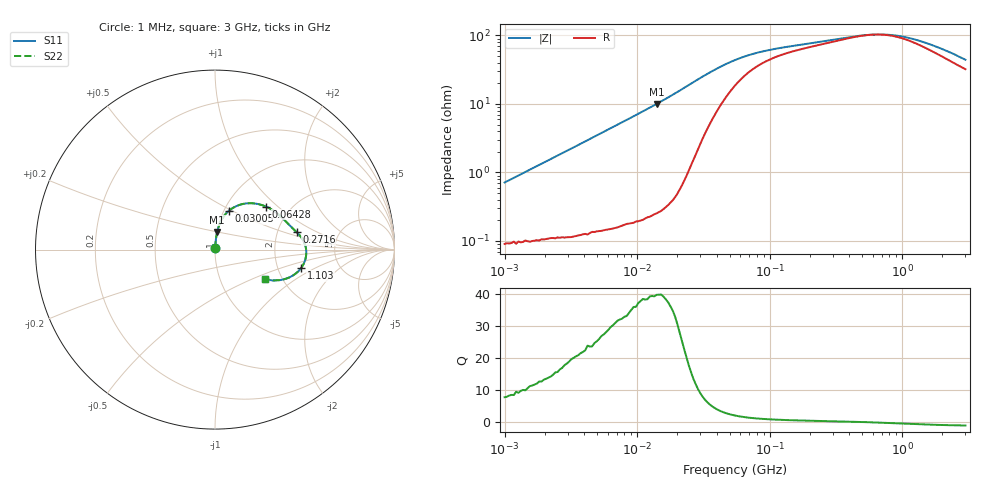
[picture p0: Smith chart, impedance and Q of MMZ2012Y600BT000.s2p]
! S-parameter Generated by TDK Corporation
! Copyright(C) 2016 TDK Corporation.
! All Rights Reserved.
! TDK P/N: MMZ2012Y600BT000 (Chip Beads)
! Property: |Z|=60¶ at 100MHz
! Size(LxWxT): 2x1.25x0.85mm, 0.079x0.049x0.033inches
! Model Type: s2p (Touchstone File Format Version 1.0)
! Frequency: DC=Yes Start=1MHz Stop=3000MHz 202points Log-sweep
! Note: This model was converted from impedance.
! Model Generated on May. 16, 2016
! Hash(MD5):
! Port Assignments:
!  1 ---@@@--- 2
! Applicable Conditions:
!  Temperature = 25 degC
!  DC Bias Current = 0 A
!  Small Signal Operation
! Terms and conditions regarding TDK Simulation Models
! (1)This simulation model is being provided solely for informational purposes. Please refer to the specifications of the products in terms of detailed characteristics of such products.
! (2)In no event shall TDK Corporation of any of its subsidiaries be liable for any loss or damage arising, directly or indirectly,
!  From any information contained in this simulation model, including, but not limited to loss or damages arising from any inaccuracies, omissions or errors in connection with such information.
! (3)Any and all copyrights on this simulation model are owned by TDK Corporation.
!  Duplication or redistribution of this simulation model without prior written permission from TDK Corporation is prohibited.
! (4)This simulation model is subject to any modification or change without any prior notice.
! (5)Neither TDK Corporation nor any of its subsidiaries shall make any warranty, express or implied,
!  Including but not limited to the correctness, implied warranties of merchantability and fitness for a particular purpose with respect to this simulation models.
! (6)The use of this simulation model shall be deemed to have consented to the terms and conditions hereof.
# MHz S MA R 50
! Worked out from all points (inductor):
!   201 points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, 1 MHz to 3 GHz, reference 50 ohm
!   read as one part in series: L = 112 nH near 1.041 MHz
!   highest Q = 39.6 at 14.04 MHz (marker M1), where L = 114 nH
!   self-resonance near 613.8 MHz
!   S11 on the Smith chart (normalised r, x): 1 MHz: 1.00, +0.01; 30.05 MHz: 1.05, +0.48; 64.28 MHz: 1.51, +0.84; 271.6 MHz: 2.55, +0.64; 1.103 GHz: 2.71, -0.72; 3 GHz: 1.64, -0.61
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1  0.007123 82.3  0.9991 -0.4  0.9991 -0.4  0.007123 82.3
3.900413  0.02729 85.8  0.9984 -1.6  0.9984 -1.6  0.02729 85.8
8.017732  0.056 85.0  0.9967 -3.2  0.9967 -3.2  0.056 85.0
14.04268  0.09951 82.8  0.9925 -5.7  0.9925 -5.7  0.09951 82.8
14.61624  0.1038 82.6  0.992 -6.0  0.992 -6.0  0.1038 82.6
21.81181  0.1612 78.5  0.9806 -9.3  0.9806 -9.3  0.1612 78.5
30.0453  0.2282 70.5  0.9487 -13.1  0.9487 -13.1  0.2282 70.5
41.38676  0.2994 58.3  0.8802 -16.8  0.8802 -16.8  0.2994 58.3
54.77226  0.3503 46.4  0.7998 -18.5  0.7998 -18.5  0.3503 46.4
64.28402  0.3715 40.2  0.7554 -18.5  0.7554 -18.5  0.3715 40.2
81.73662  0.3947 32.4  0.6997 -17.6  0.6997 -17.6  0.3947 32.4
103.9275  0.4112 26.5  0.6579 -16.2  0.6579 -16.2  0.4112 26.5
213.6344  0.4501 15.0  0.5772 -11.7  0.5772 -11.7  0.4501 15.0
271.6345  0.4648 12.2  0.5544 -10.2  0.5544 -10.2  0.4648 12.2
389.4533  0.488 7.5  0.5201 -7.0  0.5201 -7.0  0.488 7.5
536.4635  0.504 2.4  0.4968 -2.4  0.4968 -2.4  0.504 2.4
800.5644  0.5076 -5.2  0.4966 5.3  0.4966 5.3  0.5076 -5.2
1102.76  0.4913 -11.9  0.529 11.0  0.529 11.0  0.4913 -11.9
1402.151  0.4663 -17.0  0.5706 13.8  0.5706 13.8  0.4663 -17.0
1855.641  0.4244 -22.6  0.6299 15.0  0.6299 15.0  0.4244 -22.6
2455.801  0.3713 -27.6  0.6927 14.4  0.6927 14.4  0.3713 -27.6
3000  0.3261 -30.4  0.7374 12.9  0.7374 12.9  0.3261 -30.4
